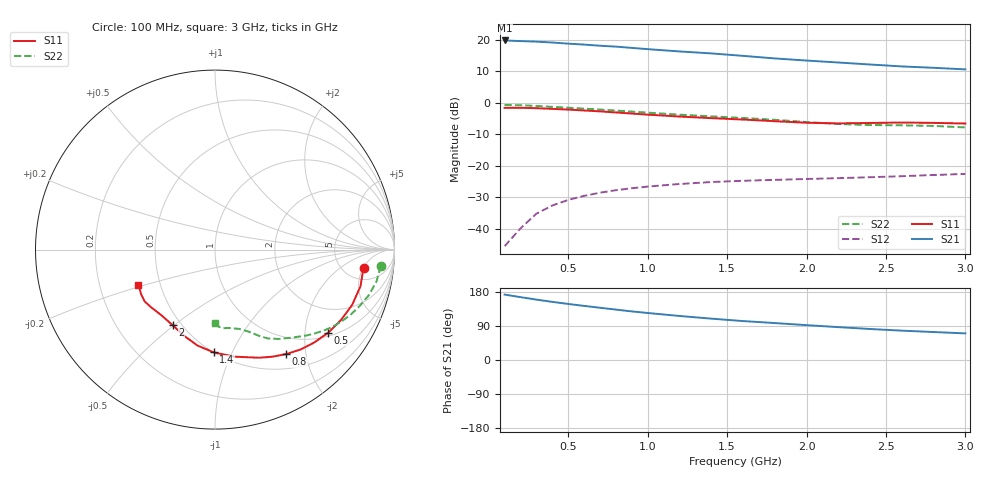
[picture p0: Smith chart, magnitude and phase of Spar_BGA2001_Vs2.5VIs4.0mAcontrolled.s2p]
! Filename: 2_54G1.001
! Title: BGA2001 X0297-20 HFE=80
! Bias: Vce=2.5V; Ic=4.0mA controlled / noise data included
! Company: NXP Semiconductors NL
! User: Quality&Reliability T&D
! Measure time: 23 Oct 1998 / 08:33:48
#  MHz  S  MA  R 50
! Freq  S11  S21  S12  S22  :
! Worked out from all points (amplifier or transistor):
!   20 points, 100 MHz to 3 GHz, reference 50 ohm
!   highest |S21| = 19.9 dB at 100 MHz (marker M1)
!   |S21| within 3 dB of that: start of sweep to 1.064 GHz
!   unconditionally stable (mu >= 1): 2.126 GHz to end of sweep
!   at 400 MHz: K = 0.21, MSG = 25.9 dB, |S12| = -32.7 dB
!   at 1.2 GHz: K = 0.53, MSG = 21.1 dB, |S12| = -25.8 dB
!   at 3 GHz: K = 1.22, MAG = 13.8 dB, |S12| = -22.6 dB
!   lowest NFmin = 1.22 dB at 1.8 GHz
!   S11 on the Smith chart (normalised r, x): 100 MHz: 7.68, -5.03; 500 MHz: 1.11, -2.64; 800 MHz: 0.72, -1.66; 1.4 GHz: 0.50, -0.85; 2 GHz: 0.45, -0.49; 3 GHz: 0.38, -0.19
100  0.8336 -6.9  9.855 172.6  0.005249 58.5  0.9282 -5.6
200  0.836 -14.1  9.63 165.9  0.01008 80.3  0.9171 -11.1
300  0.824 -21.9  9.435 159.4  0.01725 79.3  0.8945 -16.4
400  0.8041 -29.3  9.143 153.4  0.0233 74.6  0.8657 -21.2
500  0.7826 -36.2  8.767 147.9  0.02856 70.5  0.8385 -25.6
600  0.7579 -43.0  8.477 142.8  0.03315 66.9  0.8109 -29.6
700  0.7333 -49.3  8.127 137.9  0.03725 63.8  0.7837 -33.2
800  0.7043 -55.7  7.861 133.0  0.04083 60.9  0.7555 -36.7
900  0.677 -61.8  7.511 128.2  0.04382 58.5  0.7276 -39.8
1000  0.6508 -67.8  7.166 124.1  0.0466 56.5  0.7002 -43.0
1200  0.6066 -79.6  6.592 116.2  0.0512 53.0  0.6496 -49.1
1400  0.5726 -90.8  6.134 109.1  0.05503 50.4  0.6104 -54.6
1600  0.5434 -100.3  5.606 102.8  0.05762 49.0  0.5757 -59.3
1800  0.5115 -109.3  5.102 97.5  0.05959 49.0  0.5383 -63.1
2000  0.4829 -119.2  4.723 92.0  0.06154 48.2  0.4962 -67.4
2200  0.4722 -129.5  4.394 86.8  0.06349 47.6  0.4615 -73.2
2400  0.4793 -137.8  4.084 81.8  0.06564 48.0  0.4441 -79.5
2600  0.4869 -143.7  3.806 77.4  0.06814 49.5  0.4402 -84.2
2800  0.4805 -149.0  3.619 73.8  0.07128 50.0  0.4304 -87.1
3000  0.4698 -155.3  3.415 70.2  0.074 50.9  0.4068 -90.1
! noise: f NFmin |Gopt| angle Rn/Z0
900  1.25  0.38  19.1  0.29
1000  1.29  0.36  15.6  0.29
1800  1.222  0.331  64.56  0.233
2000  1.246  0.303  72.5  0.251
2200  1.402  0.246  83.7  0.215
2400  1.526  0.227  96.28  0.203
